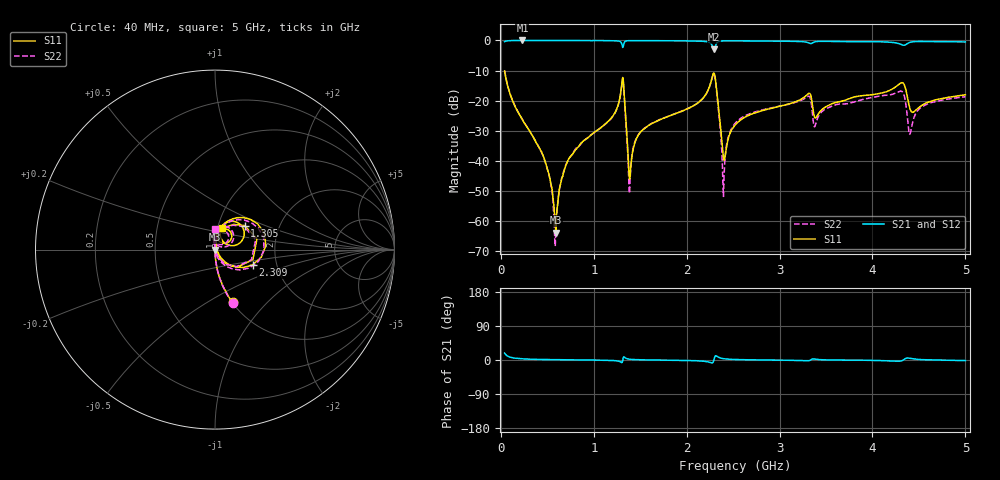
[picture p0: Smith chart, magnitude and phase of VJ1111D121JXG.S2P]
! VJ1111D121JXG
! DATE 02/15/2022  13:11
! CAPACITORS MOUNTED IN SERIES ON 25 MIL THICK MICROSTRIP SUBSTRATE
# GHz  S  MA  R  50.00
!  FREQ  S11M  S11A  S21M  S21A  S12M  S12A  S22M  S22A
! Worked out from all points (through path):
!   801 points, 40 MHz to 5 GHz, reference 50 ohm
!   highest |S21| = -0.01 dB at 232.2 MHz (marker M1); lowest = -3.0 dB at 2.297 GHz (marker M2)
!   lowest |S11| = -63.9 dB at 591.8 MHz (marker M3), VSWR 1.00, Z = 50.1 + j0.0365 ohm
!   |S11| at or under -10 dB: start of sweep to end of sweep
!   |S22| runs from -68.4 to -10.0 dB; largest |S21 - S12| = 0.0092
!   S11 on the Smith chart (normalised r, x): 40 MHz: 1.00, -0.65; 1.305 GHz: 1.34, +0.37; 2.309 GHz: 1.50, -0.27; 5 GHz: 1.05, +0.25
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0.04  0.3102 -71.5  0.9515 18.1  0.9507 18.2  0.3152 -71.5
0.2322  0.04761 -86.8  0.9991 3.1  0.9984 3.0  0.04825 -87.1
0.474  0.009935 -87.1  0.9979 1.2  1 1.3  0.009787 -88.5
0.5918  0.0006415 34.6  0.9968 0.8  1.001 0.9  0.0008041 51.4
0.6848  0.007132 81.5  0.9969 0.6  0.9996 0.5  0.00732 86.2
0.8708  0.02001 85.0  0.9951 0.2  0.9994 0.1  0.02001 88.2
1.1994  0.05389 82.7  0.9892 -1.3  0.9939 -1.4  0.05312 84.0
1.3048  0.2122 39.0  0.8378 -6.7  0.8416 -6.7  0.2061 38.6
1.3916  0.005762 46.3  0.992 1.9  0.9961 1.8  0.005152 72.5
1.4722  0.02565 85.3  0.9923 0.7  0.9976 0.7  0.02624 89.9
1.6954  0.04677 85.7  0.9899 -0.2  0.9943 -0.2  0.04721 88.3
2.2968  0.2844 4.7  0.7112 3.9  0.7143 3.8  0.2734 -0.7
2.3092  0.226 -22.0  0.8024 10.9  0.8064 10.8  0.2151 -28.7
2.396  0.01092 -5.9  0.9839 3.6  0.9879 3.5  0.002556 173.5
2.52  0.03899 82.4  0.9846 1.3  0.9893 1.3  0.04172 98.1
3.3012  0.1279 64.8  0.9249 -2.1  0.9293 -2.3  0.1169 69.0
3.3508  0.09079 29.1  0.9043 2.5  0.9084 2.3  0.06851 31.0
4.1754  0.1457 71.1  0.9369 -2.4  0.9427 -2.5  0.1236 80.2
4.3242  0.1978 39.7  0.8381 -1.0  0.8423 -1.3  0.1386 44.5
4.4048  0.07229 23.2  0.9316 4.4  0.9361 4.2  0.02796 67.0
4.5474  0.08652 70.6  0.9602 0.8  0.9649 0.6  0.0814 99.4
5  0.1248 72.9  0.9448 -1.4  0.9495 -1.6  0.1158 91.2
